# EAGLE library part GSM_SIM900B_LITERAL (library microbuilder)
SIM900B GSM/GPRS Module Supply: 3.1-4.8V Quad-Band: GSM 850, EGSM 900, DCS 1800, PCS 1900
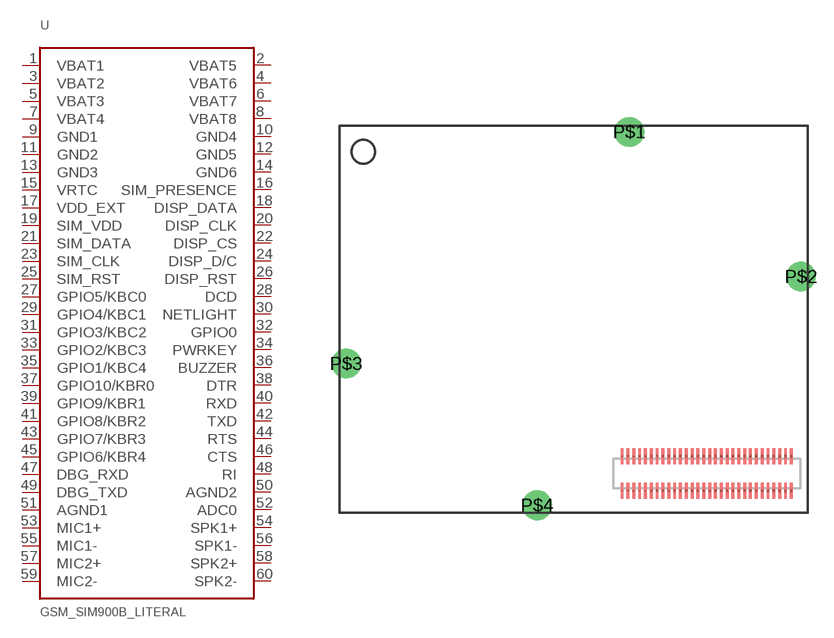
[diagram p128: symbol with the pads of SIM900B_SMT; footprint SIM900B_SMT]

Designator prefix U

## GSM_SIM900B_LITERAL  [SIM900B_SMT]
1  VBAT1  pwr
2  VBAT5  pwr
3  VBAT2  pwr
4  VBAT6  pwr
5  VBAT3  pwr
6  VBAT7  pwr
7  VBAT4  pwr
8  VBAT8  pwr
9  GND1  pwr
10  GND4  pwr
11  GND2  pwr
12  GND5  pwr
13  GND3  pwr
14  GND6  pwr
15  VRTC  pwr
16  SIM_PRESENCE  in
17  VDD_EXT  pwr
18  DISP_DATA
19  SIM_VDD  pwr
20  DISP_CLK  out
21  SIM_DATA
22  DISP_CS  out
23  SIM_CLK  out
24  DISP_D/C  out
25  SIM_RST  out
26  DISP_RST  out
27  GPIO5/KBC0  out
28  DCD  out
29  GPIO4/KBC1
30  NETLIGHT  out
31  GPIO3/KBC2
32  GPIO0
33  GPIO2/KBC3
34  PWRKEY  in
35  GPIO1/KBC4
36  BUZZER  out
37  GPIO10/KBR0  in
38  DTR  in
39  GPIO9/KBR1
40  RXD  in
41  GPIO8/KBR2
42  TXD  out
43  GPIO7/KBR3
44  RTS  in
45  GPIO6/KBR4
46  CTS  out
47  DBG_RXD  in
48  RI  out
49  DBG_TXD  out
50  AGND2  pwr
51  AGND1  pwr
52  ADC0  in
53  MIC1+  in
54  SPK1+  out
55  MIC1-  in
56  SPK1-  out
57  MIC2+  in
58  SPK2+  out
59  MIC2-  in
60  SPK2-  out

## Footprint SIM900B_SMT (pad centres in mm)
SIM900B - 60 Pin B2B Connector
smd 0.25 x 1.35: 1 -7.25,-1.475; 2 -7.25,1.475; 3 -6.75,-1.475; 4 -6.75,1.475; 5 -6.25,-1.475; 6 -6.25,1.475; 7 -5.75,-1.475; 8 -5.75,1.475; 9 -5.25,-1.475; 10 -5.25,1.475; 11 -4.75,-1.475; 12 -4.75,1.475; 13 -4.25,-1.475; 14 -4.25,1.475; 15 -3.75,-1.475; 16 -3.75,1.475; 17 -3.25,-1.475; 18 -3.25,1.475; 19 -2.75,-1.475; 20 -2.75,1.475; 21 -2.25,-1.475; 22 -2.25,1.475; 23 -1.75,-1.475; 24 -1.75,1.475; 25 -1.25,-1.475; 26 -1.25,1.475; 27 -0.75,-1.475; 28 -0.75,1.475; 29 -0.25,-1.475; 30 -0.25,1.475; 31 0.25,-1.475; 32 0.25,1.475; 33 0.75,-1.475; 34 0.75,1.475; 35 1.25,-1.475; 36 1.25,1.475; 37 1.75,-1.475; 38 1.75,1.475; 39 2.25,-1.475; 40 2.25,1.475; 41 2.75,-1.475; 42 2.75,1.475; 43 3.25,-1.475; 44 3.25,1.475; 45 3.75,-1.475; 46 3.75,1.475; 47 4.25,-1.475; 48 4.25,1.475; 49 4.75,-1.475; 50 4.75,1.475; 51 5.25,-1.475; 52 5.25,1.475; 53 5.75,-1.475; 54 5.75,1.475; 55 6.25,-1.475; 56 6.25,1.475; 57 6.75,-1.475; 58 6.75,1.475; 59 7.25,-1.475; 60 7.25,1.475
drill 1.5 pad 2.54: P$1 -6.63,29.25; P$2 8.09,16.86; P$3 -30.89,9.41; P$4 -14.53,-2.72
